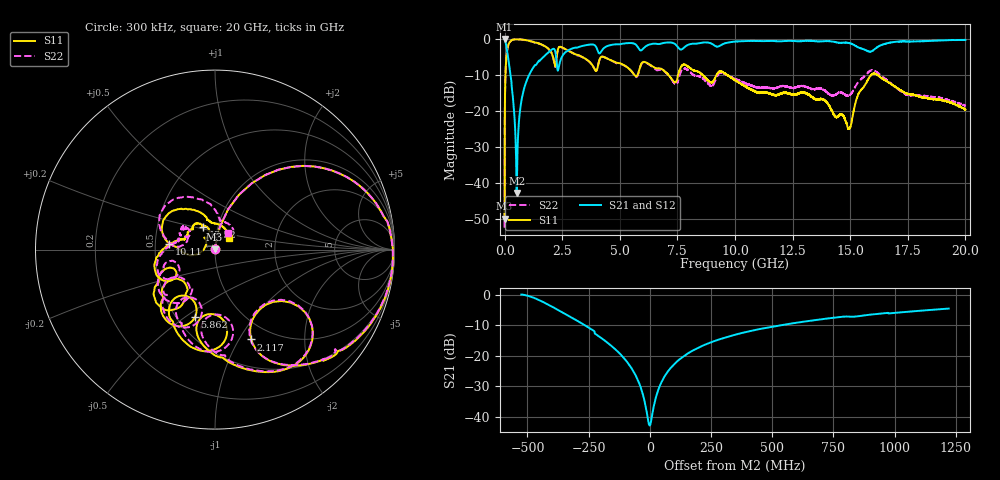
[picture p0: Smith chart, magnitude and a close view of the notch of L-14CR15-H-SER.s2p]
!{L-14CR15}
!Johanson Technology Inc.
!www.johansontechnology.com
!Test Board Conditions:
!Substrate Type  RO4350B
!Substrate Thickness  20 mil
!Substrate Dk  3.66
!TL Type: GCPW
!TL Trace Width  36 mil
!TL Gap  12 mil
!Electrode orientation  Horizontal
!DUT TOPOLOGY	SERIES
!Mounting Pad LxW  26x36 mil
! Created Sun Jun 20 13:11:08 2021
# hz S ma R 50
! 2 Port Network Data from SP1.SP block
! freq  magS11  angS11  magS21  angS21  magS12  angS12  magS22  angS22
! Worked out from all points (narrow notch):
!   20001 points, 300 kHz to 20 GHz, reference 50 ohm
!   highest |S21| = 0.00 dB at 1.3 MHz (marker M1); lowest = -42.9 dB at 525.3 MHz (marker M2)
!   notch at M2: 41.7 dB deep, 204 MHz wide at half that depth
!   lowest |S11| = -50.0 dB at 300 kHz (marker M3), VSWR 1.01, Z = 49.8 + j0.2 ohm
!   |S11| at or under -10 dB: 8.594 GHz to 9.199 GHz (604.1 MHz wide, 6.79 % of centre); 9.657 GHz to 15.91 GHz (6.252 GHz wide, 48.9 % of centre); 16.17 GHz to end of sweep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
!   |S22| runs from -52.5 to -0.1 dB; largest |S21 - S12| = 0.013
!   S11 on the Smith chart (normalised r, x): 300 kHz: 1.00, +0.00; 2.117 GHz: 0.80, -1.13; 5.862 GHz: 0.61, -0.55; 10.11 GHz: 0.59, +0.04; 13.52 GHz: 0.85, +0.22; 20 GHz: 1.16, +0.16
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300000  0.00316 140.5  0.9984 0.1  0.997 -0.1  0.002361 140.4
1300000  0.01429 89.4  0.9996 -0.7  0.9996 -0.7  0.01446 89.1
1.263e8  0.7459 37.9  0.6302 -49.6  0.6316 -49.4  0.7471 37.7
2.773e8  0.9465 13.6  0.284 -74.0  0.2848 -73.9  0.9464 13.4
5.253e8  0.9932 -5.2  0.007168 -1.0  0.007174 -0.0  0.9924 -5.3
7.313e8  0.9857 -15.1  0.1393 72.5  0.1394 72.5  0.9835 -15.3
9.673e8  0.9622 -25.2  0.2683 64.3  0.2682 64.1  0.958 -25.4
1.7223e9  0.805 -53.2  0.579 35.7  0.5804 35.6  0.7998 -53.2
2.1173e9  0.5397 -68.1  0.7327 9.0  0.734 9.1  0.5338 -68.3
2.3543e9  0.7685 -47.7  0.4081 19.3  0.4079 19.3  0.765 -47.4
3.3343e9  0.5718 -92.6  0.7962 -4.1  0.7962 -4.1  0.5677 -90.3
3.9393e9  0.3664 -97.7  0.8047 -27.3  0.8043 -27.3  0.3671 -93.5
5.8623e9  0.3927 -106.5  0.7076 -53.6  0.7079 -53.6  0.3832 -101.9
6.6673e9  0.3903 -137.0  0.853 -58.0  0.8544 -57.9  0.3688 -136.6
1.00003e10  0.268 175.9  0.9222 -100.2  0.9222 -100.2  0.2812 -179.7
1.01093e10  0.2561 173.3  0.9278 -102.2  0.9285 -102.1  0.2711 178.3
1.33343e10  0.157 117.7  0.9444 -149.0  0.943 -149.0  0.201 143.3
1.35243e10  0.1427 118.4  0.9351 -151.7  0.9285 -151.7  0.2038 145.6
1.49513e10  0.05639 159.3  0.8792 -174.0  0.8801 -174.1  0.1622 164.3
1.58933e10  0.3118 160.9  0.6682 -174.4  0.6697 -174.5  0.3649 145.5
1.66673e10  0.2481 117.5  0.8843 -179.9  0.8837 -179.1  0.2582 96.9
2e10  0.1044 39.7  0.9727 130.4  0.9723 130.4  0.1161 52.4
